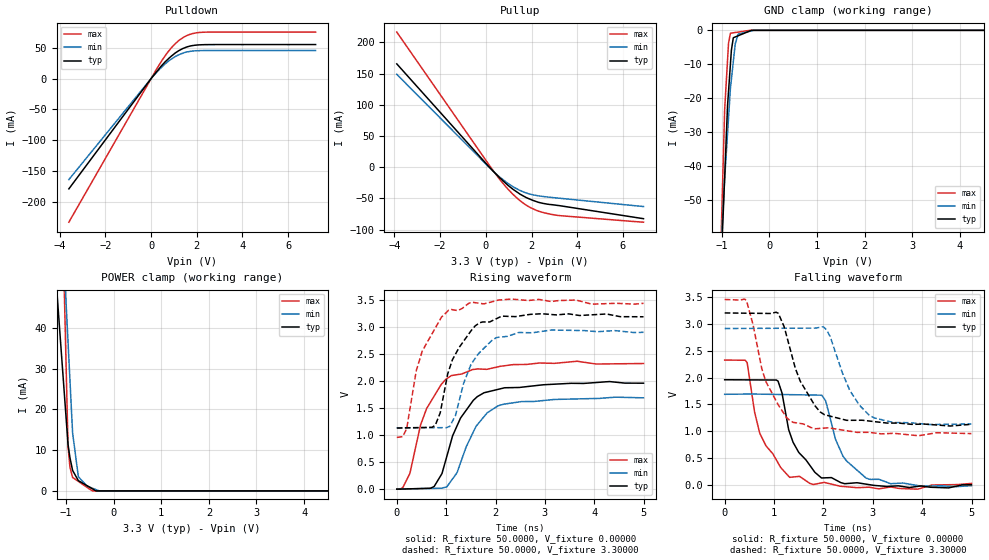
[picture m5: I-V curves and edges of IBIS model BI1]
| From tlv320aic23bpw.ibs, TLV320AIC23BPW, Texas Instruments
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[Model] BI1
Model_type I/O
Vref=0.00000V
Rref=1.00000Gohms
Cref=20.0000pF
Vmeas=1.65000V
Vinl = 990.000mV
Vinh = 2.31000V
C_comp 2.00000pF 2.00000pF 2.00000pF
| variable typ   min   max
[Voltage Range] 3.30000V 3.00000V 3.60000V
[POWER Clamp Reference] 3.30000V 3.00000V 3.60000V
[Pullup Reference] 3.30000V 3.00000V 3.60000V
[Pulldown Reference] 0.00000V 0.00000V 0.00000V
[GND Clamp Reference] 0.00000V 0.00000V 0.00000V
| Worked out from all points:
|   slope of the pulldown table from 0 to 0.495 V, typ, clamps not added: 22.1 ohm
|   slope of the pullup table from 0 to 0.495 V, typ, clamps not added: 25.9 ohm
|   GND clamp passes 1 mA (typ) near -0.55 V on its own axis
|   POWER clamp passes 1 mA (typ) near -0.52 V on its own axis
|   rising waveform, R_fixture 50.0000, V_fixture 0.00000: 20-80 % time 543ps typ, 543ps min, 541ps max; typ from 0 V to 1.97 V
|   falling waveform, R_fixture 50.0000, V_fixture 0.00000: 20-80 % time 512ps typ, 511ps min, 510ps max; typ from 1.96 V to 0.013 V
|   falling waveform, R_fixture 50.0000, V_fixture 3.30000: 20-80 % time 532ps typ, 514ps min, 529ps max; typ from 3.2 V to 1.13 V
|   rising waveform, R_fixture 50.0000, V_fixture 3.30000: 20-80 % time 478ps typ, 477ps min, 495ps max; typ from 1.13 V to 3.2 V
[GND Clamp]
-3.6V     -1.17A     -748.3mA   -1.371A
-1.003V   -64.49mA   -59.98mA   -54.23mA
-941.8mV  -43.34mA   -43.87mA   -23.43mA
-881mV    -22.18mA   -30.42mA   -8.736mA
-860.8mV  -18.09mA   -25.95mA   -3.844mA
-820.5mV  -9.938mA   -17.04mA   -853.1uA
-800.3mV  -5.859mA   -14.44mA   -811.1uA
-759.9mV  -2.183mA   -9.226mA   -727.1uA
-719.4mV  -1.951mA   -4.009mA   -642.9uA
-658.7mV  -1.602mA   -1.133mA   -516.7uA
-329.4mV  0A         0A         0A
7.2V      0A         0A         0A
[Pulldown]
-3.6V     -178.8mA   -163.8mA   -232.9mA
238.5mV   10.93mA    9.835mA    15.35mA
719.2mV   30.77mA    27mA       42.27mA
880.9mV   36.2mA     31.51mA    49.68mA
1.219V    45.35mA    38.72mA    61.86mA
1.422V    49.17mA    41.64mA    67.05mA
1.679V    52.47mA    43.88mA    71.45mA
2.18V     54.78mA    45.35mA    74.93mA
7.2V      55.12mA    45.55mA    75.36mA
[Pullup]
-3.9V     165.5mA    148.8mA    216.4mA
300mV     -5.49mA    -5.77mA    -4.496mA
917.5mV   -27.27mA   -24.61mA   -33.04mA
1.52V     -43.58mA   -37.65mA   -54.3mA
1.817V    -49.35mA   -41.83mA   -61.93mA
2.257V    -55.59mA   -45.53mA   -69.72mA
2.879V    -59.91mA   -48.38mA   -75.5mA
6.9V      -82.37mA   -62.92mA   -87.97mA
[POWER Clamp]
-3.9V     483.1mA    720.2mA    1.742A
-1.201V   50.29mA    92.89mA    128.9mA
-958.3mV  11.4mA     36.54mA    10.94mA
-917.8mV  8.133mA    27.13mA    5.782mA
-862.1mV  5.014mA    14.18mA    3.305mA
-741.1mV  2.525mA    3.47mA     2.334mA
-559.1mV  1.285mA    1.188mA    872.7uA
-442.4mV  489.5uA    651.8uA    0A
-370.6mV  0A         321.8uA    0A
-301mV    0A         2.297uA    0A
6.9V      0A         0A         0A
[Rising Waveform]
R_fixture = 50.0000
V_fixture = 0.00000
V_fixture_min = 0.00000
V_fixture_max = 0.00000
0s        379.2uV    582.9uV    899.3uV
125ps     3.446mV    3.044mV    33.79mV
265ps     6.881mV    5.801mV    291.4mV
480ps     12.16mV    10.03mV    1.187V
755ps     48.17mV    15.45mV    1.724V
915ps     288.9mV    19.78mV    1.958V
1.105ns   907.9mV    159.8mV    2.107V
1.55ns    1.648V     1.062V     2.22V
2.05ns    1.851V     1.546V     2.269V
4.995ns   1.965V     1.694V     2.33V
[Falling Waveform]
R_fixture = 50.0000
V_fixture = 0.00000
V_fixture_min = 0.00000
V_fixture_max = 0.00000
0s        1.959V     1.689V     2.324V
455ps     1.956V     1.694V     2.276V
605ps     1.956V     1.693V     1.359V
710ps     1.955V     1.692V     967.1mV
1.08ns    1.934V     1.686V     418mV
1.315ns   980.7mV    1.683V     149.5mV
1.965ns   137.9mV    1.673V     47.29mV
2.395ns   40.6mV     540.9mV    -19.42mV
2.865ns   23.03mV    133.8mV    -35.41mV
4.995ns   12.72mV    -4.793mV   37.09mV
[Falling Waveform]
R_fixture = 50.0000
V_fixture = 3.30000
V_fixture_min = 3.00000
V_fixture_max = 3.60000
0s        3.197V     2.909V     3.447V
445ps     3.192V     2.91V      3.415V
835ps     3.188V     2.912V     1.922V
1.085ns   3.191V     2.913V     1.493V
1.335ns   2.495V     2.914V     1.191V
1.53ns    1.932V     2.915V     1.149V
2.02ns    1.311V     2.921V     1.063V
2.535ns   1.207V     1.757V     1.004V
2.935ns   1.192V     1.293V     982.1mV
4.995ns   1.133V     1.139V     960.5mV
[Rising Waveform]
R_fixture = 50.0000
V_fixture = 3.30000
V_fixture_min = 3.00000
V_fixture_max = 3.60000
0s        1.133V     1.139V     960.5mV
200ps     1.137V     1.139V     1.121V
395ps     1.141V     1.14V      2.199V
780ps     1.186V     1.14V      2.988V
880ps     1.417V     1.141V     3.15V
1.05ns    2.19V      1.158V     3.318V
1.19ns    2.506V     1.372V     3.318V
1.505ns   2.939V     2.317V     3.46V
2.02ns    3.163V     2.813V     3.497V
4.995ns   3.197V     2.909V     3.447V
[Ramp]
| variable typ min max
dV/dt_r 1.17499/528.096p 1.01293/529.175p 1.39376/523.387p
dV/dt_f 1.23835/526.600p 1.06193/508.081p 1.49166/535.091p
R_load = 50.0000Ohms
